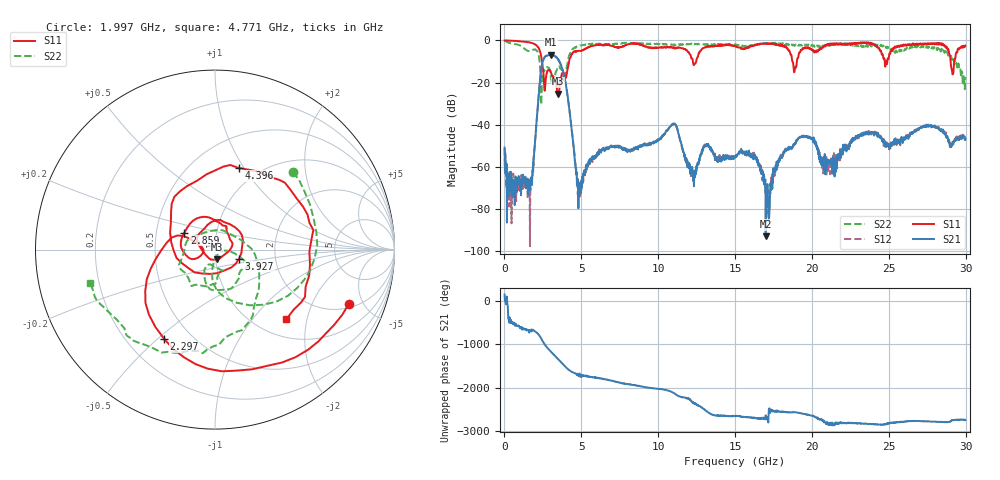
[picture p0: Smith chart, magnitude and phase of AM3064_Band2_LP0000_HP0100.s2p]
# Hz S DB R 50.0
!freq dBS11 angS11 dBS21 angS21 dBS12 angS12 dBS22 angS22
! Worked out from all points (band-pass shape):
!   1600 points, 10 MHz to 29.98 GHz, reference 50 ohm
!   highest |S21| = -6.84 dB at 3.009 GHz (marker M1); lowest = -92.9 dB at 16.99 GHz (marker M2)
!   |S21| within 3 dB of the highest: 2.501 GHz to 3.549 GHz (1.048 GHz wide, 34.7 % of centre)
!   lowest |S11| = -25.3 dB at 3.478 GHz (marker M3), VSWR 1.12, Z = 51 - j5.42 ohm
!   |S11| at or under -10 dB: 2.437 GHz to 4.205 GHz (1.768 GHz wide, 53.2 % of centre); 18.73 GHz to 19.02 GHz (288.9 MHz wide, 1.53 % of centre); 29.02 GHz to 29.25 GHz (227.2 MHz wide, 0.78 % of centre)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
!   |S22| runs from -30.5 to -0.2 dB; largest |S21 - S12| = 0.015
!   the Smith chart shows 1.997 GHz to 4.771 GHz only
!   S11 on the Smith chart (normalised r, x): 1.997 GHz: 2.26, -3.87; 2.297 GHz: 0.35, -0.53; 2.859 GHz: 0.70, +0.14; 3.927 GHz: 1.30, -0.13; 4.396 GHz: 0.81, +0.95; 4.771 GHz: 1.34, -1.51
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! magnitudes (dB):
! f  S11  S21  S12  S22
! 10 MHz  0.0  -50.8  -51.1  -0.2
! 347.4 MHz  -0.1  -71.7  -68.3  -1.3
! 1.584 GHz  -0.9  -66.9  -67.7  -5.1
! 1.997 GHz  -1.9  -47.5  -47.2  -4.2
! 2.297 GHz  -4.8  -20.1  -20.1  -11.2
! 2.859 GHz  -14.2  -7.1  -7.0  -12.9
! 3.009 GHz  -14.8  -6.8  -6.8  -16.9
! 3.478 GHz  -25.3  -8.8  -8.9  -13.5
! 3.927 GHz  -16.8  -18.6  -18.3  -18.7
! 4.396 GHz  -6.5  -43.8  -43.7  -4.7
! 4.771 GHz  -5.1  -66.4  -73.2  -2.9
! 5.015 GHz  -4.9  -70.1  -70.7  -2.4
! 6.308 GHz  -2.0  -51.9  -52.4  -1.6
! 10 GHz  -3.4  -47.5  -47.5  -1.7
! 11.09 GHz  -3.9  -39.5  -39.7  -2.0
! 12.23 GHz  -8.7  -63.2  -62.0  -1.8
! 15 GHz  -2.6  -55.2  -54.4  -1.8
! 16.99 GHz  -1.4  -92.9  -70.6  -1.3
! 19.99 GHz  -4.2  -46.6  -46.4  -2.1
! 21.45 GHz  -2.1  -60.3  -57.0  -2.0
! 25 GHz  -8.2  -50.6  -49.4  -3.2
! 29.98 GHz  -2.4  -46.9  -47.0  -17.3
